PROGRAM p05_ST_if
VAR
	switch: BOOL;
	light: BOOL;
	button1: BOOL;
	button2: BOOL;
END_VAR

// IF statement
IF switch = TRUE THEN
	light := TRUE;
END_IF

// If the condition is not true, the light does not change state, so
// the state is preserved/memorized. Explicitly, we would write it as:
IF switch = TRUE THEN
	light := TRUE;
ELSE
	light := light;
END_IF

// Is this what we wanted? Or would we like the light to turn off
// when the switch is turned off?
IF switch THEN
	light := TRUE;
ELSE
	light := FALSE;
END_IF

// Do we even need a conditional statement for this? No ...
light := switch;

// Whenever possible, replace conditional statements with logical expressions
IF switch THEN
	IF button1 THEN
		light := TRUE;
	ELSE 
		light := FALSE;
	END_IF
ELSE
	light := button2;
END_IF

// Same as:
light := (switch AND button1) OR (NOT switch AND button2);

END_PROGRAM
